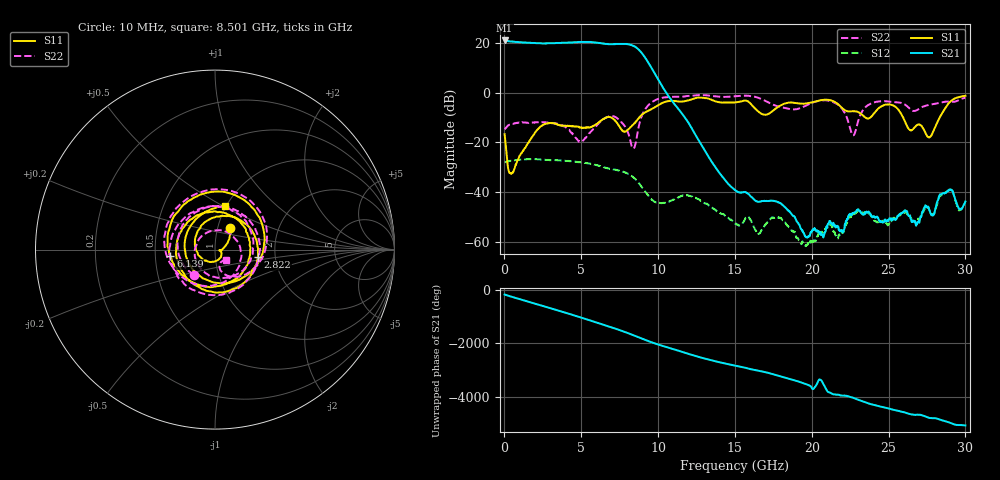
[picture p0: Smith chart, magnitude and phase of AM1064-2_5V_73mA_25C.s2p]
!Agilent	"Technologies,E8364B,MY43040894,A.07.50.67"
!Agilent	E8364B:	A.07.50.67
!Date:	"Wednesday,"	May	"01,"	2019	6:56:33
!Correction:	S11(Full	2	"Port(1,2))"
!S21(Full	2	"Port(1,2))"
!S12(Full	2	"Port(1,2))"
!S22(Full	2	"Port(1,2))"
!S2P	File:	Measurements:	"S11,"	"S21,"	"S12,"	S22:
#	Hz	S	dB	R	50
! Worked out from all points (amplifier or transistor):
!   1601 points, 10 MHz to 30 GHz, reference 50 ohm
!   highest |S21| = 20.9 dB at 10 MHz (marker M1)
!   |S21| within 3 dB of that: start of sweep to 8.613 GHz
!   unconditionally stable (mu >= 1): start of sweep to end of sweep
!   at 4.996 GHz: K = 1.38, MAG = 20.5 dB, |S12| = -28.0 dB
!   at 15.01 GHz: K = 3363.06, MAG = -31.5 dB, |S12| = -52.6 dB
!   at 30 GHz: K = 1214.35, MAG = -33.7 dB, |S12| = -44.1 dB
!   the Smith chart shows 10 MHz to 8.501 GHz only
!   S11 on the Smith chart (normalised r, x): 10 MHz: 1.15, +0.28; 2.822 GHz: 1.62, -0.14; 6.139 GHz: 0.60, -0.04; 8.501 GHz: 0.98, +0.51
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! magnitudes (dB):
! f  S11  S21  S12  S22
! 10 MHz  -16.7  20.9  -27.9  -14.7
! 459.9 MHz  -32.4  20.5  -27.3  -12.7
! 2.822 GHz  -12.3  19.8  -27.0  -12.1
! 5.015 GHz  -14.0  20.3  -28.0  -19.6
! 6.139 GHz  -12.0  19.9  -29.3  -12.3
! 7.226 GHz  -11.4  19.5  -31.0  -9.8
! 8.501 GHz  -12.0  18.4  -34.6  -21.3
! 9.063 GHz  -8.3  14.8  -38.9  -7.7
! 10.02 GHz  -5.0  5.1  -44.2  -2.5
! 12.02 GHz  -3.0  -12.6  -41.4  -1.4
! 15.01 GHz  -3.9  -39.1  -52.6  -1.5
! 16.54 GHz  -7.7  -43.8  -56.7  -2.2
! 17.84 GHz  -5.6  -44.0  -50.1  -5.6
! 20.01 GHz  -3.9  -55.4  -59.6  -4.1
! 21.17 GHz  -3.0  -51.6  -53.1  -3.4
! 21.72 GHz  -4.7  -53.8  -58.5  -4.9
! 22.69 GHz  -7.5  -48.4  -48.7  -17.1
! 23.53 GHz  -10.2  -48.1  -48.1  -5.7
! 25.01 GHz  -4.7  -51.0  -52.6  -3.6
! 27.64 GHz  -18.0  -47.0  -46.9  -5.0
! 28.97 GHz  -3.9  -39.1  -38.9  -3.6
! 30 GHz  -1.3  -43.7  -44.1  -2.1
